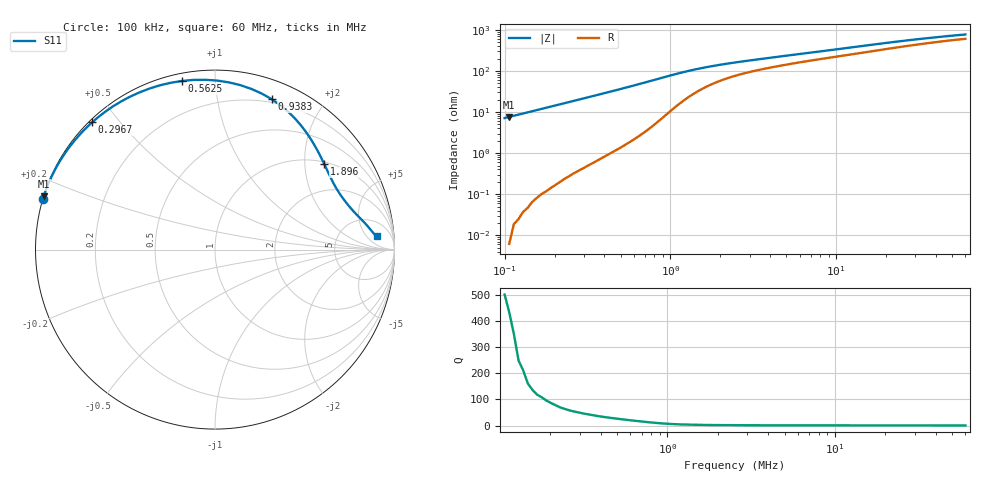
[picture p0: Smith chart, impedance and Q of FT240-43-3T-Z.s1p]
! ListType=Log
!!FT240-43 3T Z
# MHz S RI R 50
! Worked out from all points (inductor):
!   101 points, 100 kHz to 60 MHz, reference 50 ohm
!   read as one part to ground: L = 11.3 uH near 100 kHz
!   highest Q = 432 at 106.6 kHz (marker M1), where L = 11.3 uH
!   S11 on the Smith chart (normalised r, x): 100 kHz: -0.00, +0.14; 296.7 kHz: 0.01, +0.42; 562.5 kHz: 0.04, +0.82; 938.3 kHz: 0.17, +1.43; 1.896 MHz: 1.06, +2.51; 60 MHz: 12, +10
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0.1  -0.9605 0.2793
0.106606  -0.9547 0.2968
0.1376916  -0.9242 0.3771
0.1668215  -0.8896 0.4483
0.2021141  -0.8414 0.5289
0.2296993  -0.7992 0.5868
0.2610494  -0.7475 0.6472
0.2966783  -0.685 0.7088
0.3371699  -0.6103 0.7692
0.3831879  -0.5227 0.8258
0.4354866  -0.422 0.8754
0.5276177  -0.2488 0.929
0.5624719  -0.1861 0.9394
0.6392399  -0.0559 0.9462
0.7264854  0.076 0.932
0.8256385  0.203 0.8951
0.9383242  0.3166 0.8376
1.06639  0.4094 0.7664
1.136835  0.4472 0.7286
1.377343  0.531 0.6198
1.565327  0.5687 0.556
1.896486  0.6091 0.4759
2.611302  0.6555 0.3786
3.595545  0.6944 0.3121
5.626461  0.7446 0.2447
12.92394  0.8224 0.1609
27.84666  0.8711 0.1059
60  0.9002 0.0731
